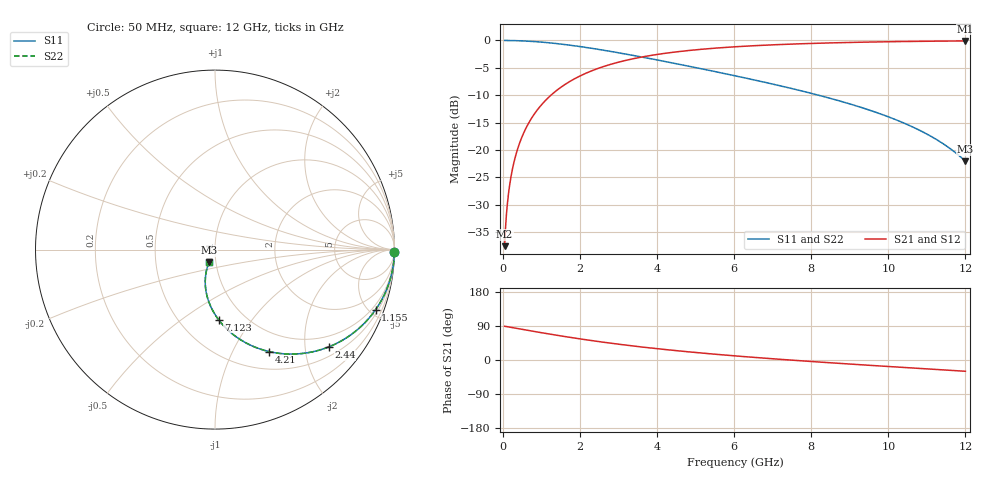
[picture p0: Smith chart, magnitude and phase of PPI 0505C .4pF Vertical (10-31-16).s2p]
# GHz S MA R 50
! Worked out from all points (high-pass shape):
!   1601 points, 50 MHz to 12 GHz, reference 50 ohm
!   highest |S21| = -0.09 dB at 12 GHz (marker M1); lowest = -37.5 dB at 50 MHz (marker M2)
!   |S21| within 3 dB of the highest: 3.56 GHz to end of sweep
!   lowest |S11| = -22.1 dB at 12 GHz (marker M3), VSWR 1.17, Z = 46.3 - j6.66 ohm
!   |S11| at or under -10 dB: 8.195 GHz to end of sweep
!   |S22| runs from -22.1 to 0.0 dB; largest |S21 - S12| = 0
!   S11 on the Smith chart (normalised r, x): 50 MHz: open; 1.155 GHz: 0.71, -5.44; 2.44 GHz: 0.71, -2.53; 4.21 GHz: 0.72, -1.40; 7.123 GHz: 0.76, -0.70; 12 GHz: 0.93, -0.13
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0.05  0.9999 -0.9  0.01326 89.1  0.01326 89.1  0.9999 -0.9
0.139625  0.9993 -2.5  0.03702 87.5  0.03702 87.5  0.9993 -2.5
0.1919063  0.9987 -3.5  0.05085 86.5  0.05085 86.5  0.9987 -3.5
0.2740625  0.9973 -5.0  0.07254 85.0  0.07254 85.0  0.9973 -5.0
0.3860938  0.9947 -7.0  0.1019 83.0  0.1019 83.0  0.9947 -7.0
0.528  0.9902 -9.5  0.1388 80.4  0.1388 80.4  0.9902 -9.5
0.6997813  0.983 -12.6  0.1828 77.4  0.1828 77.4  0.983 -12.6
0.9089063  0.9718 -16.3  0.235 73.7  0.235 73.7  0.9718 -16.3
1.155375  0.9555 -20.5  0.2941 69.5  0.2941 69.5  0.9555 -20.5
1.558688  0.9226 -27.2  0.3845 62.7  0.3845 62.7  0.9226 -27.2
2.044156  0.8757 -34.8  0.4813 55.1  0.4813 55.1  0.8757 -34.8
2.44  0.8338 -40.6  0.5502 49.3  0.5502 49.3  0.8338 -40.6
3.179406  0.7525 -50.4  0.6563 39.5  0.6563 39.5  0.7525 -50.4
4.038312  0.6604 -60.3  0.7481 29.5  0.7481 29.5  0.6604 -60.3
4.210094  0.6427 -62.1  0.7631 27.7  0.7631 27.7  0.6427 -62.1
5.091406  0.5572 -70.7  0.8269 19.0  0.8269 19.0  0.5572 -70.7
6.025  0.476 -78.7  0.8755 10.9  0.8755 10.9  0.476 -78.7
7.122906  0.391 -87.1  0.9158 2.3  0.9158 2.3  0.391 -87.1
8.019156  0.3281 -93.3  0.9396 -4.1  0.9396 -4.1  0.3281 -93.3
10.01331  0.2003 -105.7  0.9737 -17.2  0.9737 -17.2  0.2003 -105.7
11.13363  0.1318 -111.7  0.9846 -24.3  0.9846 -24.3  0.1318 -111.7
12  0.07886 -115.0  0.9896 -29.7  0.9896 -29.7  0.07886 -115.0
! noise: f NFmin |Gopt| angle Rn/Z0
0.05  0.002254  0.9868  0.8657  0.03918
1.372  0.005973  0.7934  8.793  0.005935
2.701  0.009087  0.7252  12.23  0.006496
4.031  0.01189  0.6873  15.53  0.007258
5.36  0.01455  0.6626  18.83  0.008044
6.682  0.01714  0.6458  22.1  0.008848
8.012  0.01974  0.6344  25.34  0.009697
9.341  0.0224  0.6273  28.53  0.01061
10.67  0.02515  0.6237  31.67  0.01162
12  0.02805  0.6233  34.75  0.01274
